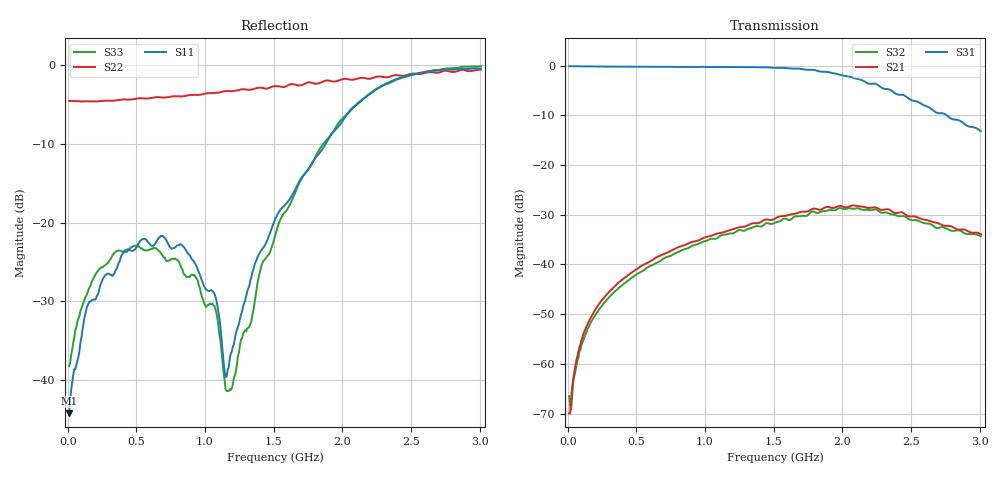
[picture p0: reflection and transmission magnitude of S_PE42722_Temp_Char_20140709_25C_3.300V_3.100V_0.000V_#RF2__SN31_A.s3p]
! Device ID: PE42722_Temp_Char_20140709
! Dir: c:\SVN\PSC 4Port_VNA Bench\CVI 2009\datafile\PE42722\PE42722_Temp_Char_20140709\25C\3p300000\#RF2
! Serial: 31
! Insertion: A
! Temp: 25C
! VDD: 3.300
! Control_Hi: 3.100
! Control_Lo: 0.000
! Logic State: #RF2
! ThroughPath: 3-1
! Port 1: RFC
! Port 2: RF1
! Port 3: RF2
! IDD: 1.181756e-04
! FILE NAME
! DATE 07/10/14  13:51
! CORRECTED  DATA
#  Hz  S  RI  R  75
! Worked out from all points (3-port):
!   401 points, 10 MHz to 3.01 GHz, reference 75 ohm
!   strongest paths, dB at 10 MHz, 760 MHz, 1.51 GHz, 2.26 GHz, 3.01 GHz:
!     S31: -0.1, -0.3, -0.5, -3.9, -13.2
!     S21: -69.9, -37.1, -30.8, -28.7, -33.9
!     S32: -66.5, -38.1, -31.6, -29.1, -34.3
!   lowest |S11| = -44.2 dB at 10 MHz (marker M1), VSWR 1.01, Z = 75.8 + j0.543 ohm
!   |S11| at or under -10 dB: start of sweep to 1.879 GHz
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1e7  0.00502 0.00358  0.00012 0.000235  0.982 -0.013
     0.000194 0.000252  -0.593 0.00526  0.000292 0.000364
     0.985 -0.0103  -2.24e-05 0.000474  0.0119 0.0032
1.15e8  0.0131 0.019  0.000275 0.00198  0.9707 -0.1207
        0.000259 0.002  -0.5863 0.0496  0.000388 0.00171
        0.9746 -0.1216  0.000408 0.00172  0.0148 0.0274
3.55e8  0.0328 0.039  0.00181 0.00599  0.9057 -0.3559
        0.00181 0.006  -0.5806 0.1425  0.00279 0.00478
        0.9085 -0.3571  0.00278 0.00475  0.0229 0.0621
8.35e8  0.0518 0.0498  0.00955 0.0121  0.6129 -0.7494
        0.00974 0.0119  -0.5742 0.2681  0.0133 0.00404
        0.6124 -0.7516  0.0133 0.00427  0.0109 0.0494
1.0675e9  0.0321 0.0157  0.0157 0.013  0.3945 -0.886
          0.0155 0.0126  -0.5792 0.3283  0.0177 -0.00183
          0.393 -0.8852  0.0181 -0.00182  0.00142 0.0297
1.1725e9  0.00866 -0.00844  0.0188 0.0122  0.279 -0.9247
          0.0185 0.0119  -0.5841 0.3551  0.0192 -0.00528
          0.2775 -0.9266  0.0197 -0.00538  -0.00221 0.00824
1.51e9  -0.0605 -0.0852  0.0295 0.00619  -0.1464 -0.9496
        0.0281 0.00661  -0.5823 0.4513  0.0175 -0.019
        -0.1512 -0.9372  0.0173 -0.0199  -0.0599 -0.0564
2.035e9  -0.4685 -0.1394  0.031 -0.023  -0.7213 -0.3788
         0.0321 -0.0197  -0.6142 0.5396  -0.0147 -0.0342
         -0.6719 -0.399  -0.0152 -0.033  -0.4689 -0.1338
2.3875e9  -0.812 0.0309  0.0103 -0.0286  -0.4906 0.0684
          0.0142 -0.0296  -0.7031 0.5035  -0.0307 -0.0091
          -0.5236 0.0166  -0.03 -0.00904  -0.8031 0.0319
3.01e9  -0.9435 0.1257  -0.000427 -0.0197  -0.184 0.1071
        -0.00275 -0.0199  -0.9159 0.1968  -0.0151 0.0124
        -0.1779 0.1273  -0.0153 0.0117  -0.9854 -0.00893
